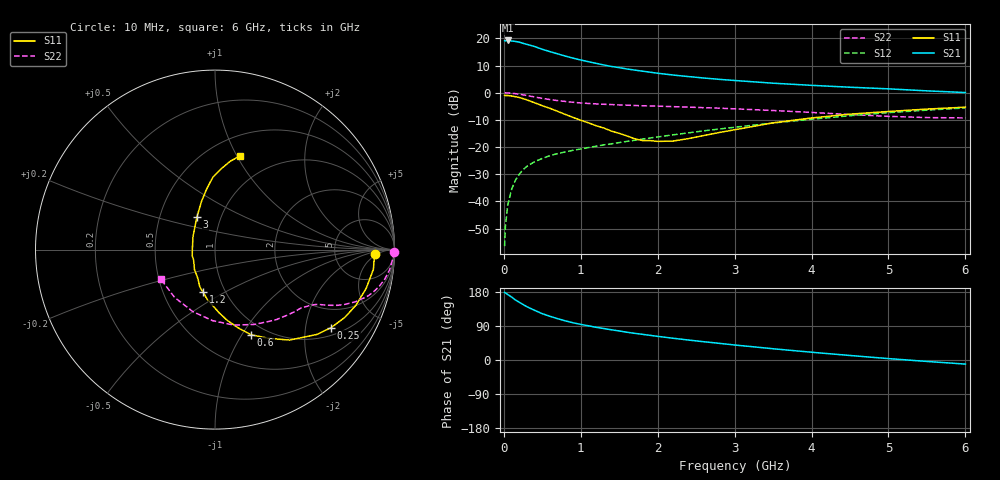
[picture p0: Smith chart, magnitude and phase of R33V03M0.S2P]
! SIEMENS Small Signal Semiconductors
! BFR181
! Si NPN RF Bipolar Junction Transistor in SOT23
! VCE = 3 V  IC = 3 mA
! Common Emitter S-Parameters:  May  1996
# GHz  S  MA  R  50
!  f  S11  S21  S12  S22
! GHz  MAG  ANG  MAG  ANG  MAG  ANG  MAG  ANG
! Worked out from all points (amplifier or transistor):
!   36 points, 10 MHz to 6 GHz, reference 50 ohm
!   highest |S21| = 19.2 dB at 50 MHz (marker M1)
!   |S21| within 3 dB of that: start of sweep to 475.2 MHz
!   unconditionally stable (mu >= 1): 1.363 GHz to 3.195 GHz
!   at 250 MHz: K = 0.30, MSG = 23.3 dB, |S12| = -28.3 dB
!   at 1.4 GHz: K = 1.01, MAG = 13.5 dB, |S12| = -18.8 dB
!   at 6 GHz: K = 0.85, MSG = 2.8 dB, |S12| = -5.6 dB
!   lowest NFmin = 1.40 dB at 450 MHz
!   S11 on the Smith chart (normalised r, x): 10 MHz: 17, -4; 250 MHz: 1.25, -2.76; 600 MHz: 0.85, -1.10; 1.2 GHz: 0.79, -0.40; 3 GHz: 0.77, +0.29; 6 GHz: 0.70, +1.03
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0.01  0.8936 -1.5  9.064 178.6  0.0015 96.5  0.9958 -0.7
0.02  0.8887 -2.8  9.015 176.9  0.0034 80.3  0.995 -1.4
0.05  0.8893 -7.1  9.156 172.9  0.0085 87.7  0.99 -3.4
0.1  0.8695 -14.4  8.96 166.2  0.0166 82.6  0.9793 -6.6
0.15  0.8449 -21.4  8.776 158.5  0.0244 77.9  0.9607 -9.8
0.2  0.8159 -27.6  8.531 152.4  0.0316 75.1  0.9386 -12.5
0.25  0.7786 -34.0  8.112 146.4  0.0383 71.3  0.9136 -15.0
0.3  0.7387 -39.8  7.757 140.6  0.0442 69.1  0.8887 -17.0
0.4  0.6532 -50.5  7.082 131.1  0.0537 65.1  0.8344 -20.4
0.5  0.5773 -58.9  6.295 122.2  0.0618 62.1  0.7865 -22.8
0.6  0.5149 -67.1  5.701 115.3  0.0696 60.1  0.7488 -24.5
0.8  0.3985 -80.4  4.717 103.3  0.0816 58.2  0.6905 -26.6
0.9  0.3511 -86.5  4.329 98.2  0.0872 58.0  0.6669 -27.4
1.1  0.2788 -99.2  3.723 90.2  0.098 58.0  0.6344 -28.9
1.2  0.247 -105.6  3.469 86.3  0.1036 58.3  0.6228 -29.7
1.6  0.1604 -135.3  2.735 73.3  0.1271 59.0  0.5903 -33.0
2.2  0.129 165.1  2.117 57.4  0.1678 59.5  0.5541 -39.7
3  0.208 118.9  1.679 39.6  0.2315 56.8  0.5054 -51.9
3.5  0.2791 105.6  1.497 29.7  0.2768 53.7  0.4705 -62.4
4.5  0.4032 91.7  1.262 11.9  0.3773 44.3  0.3965 -91.8
5.5  0.5002 80.1  1.082 -3.8  0.4783 31.9  0.3487 -130.2
6  0.5419 74.9  1.007 -10.8  0.5248 24.7  0.3436 -151.2
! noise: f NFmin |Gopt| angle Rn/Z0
0.45  1.4  0.56  17  0.36
0.9  1.5  0.45  35  0.34
1.8  1.85  0.25  82  0.36
